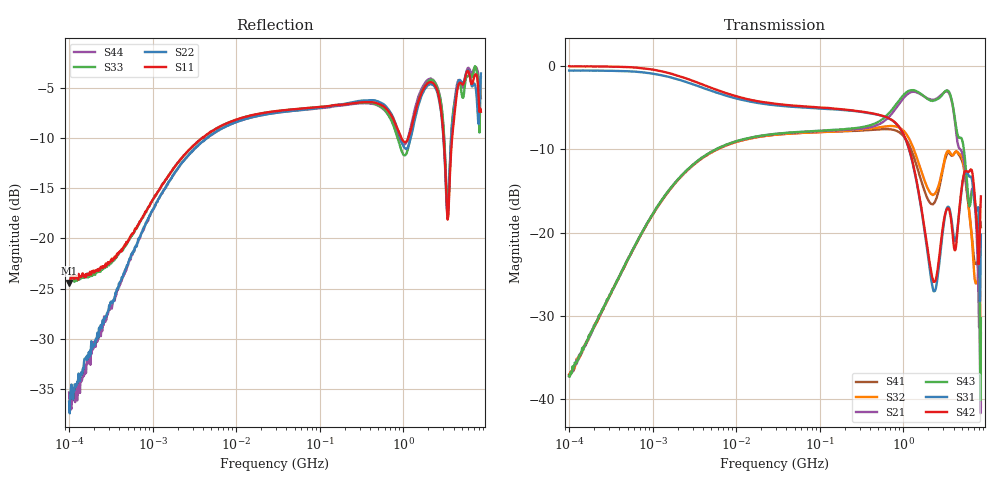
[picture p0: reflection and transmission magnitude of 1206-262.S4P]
!Agilent Technologies,E5071C,MY46110495,A.10.06
!Date: Tue Jun 06 11:35:06 2017
!Data & Calibration Information:
!Freq	S11:SOLT4(ON)	S12:SOLT4(ON)	S13:SOLT4(ON)	S14:SOLT4(ON)
!	S21:SOLT4(ON)	S22:SOLT4(ON)	S23:SOLT4(ON)	S24:SOLT4(ON)
!	S31:SOLT4(ON)	S32:SOLT4(ON)	S33:SOLT4(ON)	S34:SOLT4(ON)
!	S41:SOLT4(ON)	S42:SOLT4(ON)	S43:SOLT4(ON)	S44:SOLT4(ON)
!PortZ  Port1:50+j0  Port2:50+j0  Port3:50+j0  Port4:50+j0
!Above PortZ is port z conversion or system Z0 setting when saving the data.
!When reading, reference impedance value at option line is always used.
# Hz S dB R 50
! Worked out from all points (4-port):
!   801 points, 100 kHz to 8.5 GHz, reference 50 ohm
!   strongest paths, dB at 100 kHz, 1.721 MHz, 29.51 MHz, 502.3 MHz, 8.5 GHz:
!     S42: -0.1, -1.0, -4.6, -5.9, -15.7
!     S31: -0.6, -1.5, -4.8, -5.9, -20.2
!     S43: -37.2, -14.4, -8.2, -6.7, -30.3
!     S21: -37.2, -14.4, -8.2, -7.1, -32.0
!     S32: -37.2, -14.5, -8.3, -7.4, -40.8
!     S41: -37.0, -14.5, -8.3, -7.7, -19.4
!   lowest |S11| = -24.4 dB at 100 kHz (marker M1), VSWR 1.13, Z = 56.2 + j1.36 ohm
!   |S11| at or under -10 dB: start of sweep to 3.936 MHz; 947.3 MHz to 1.151 GHz (203.9 MHz wide, 19.4 % of centre); 3.04 GHz to 3.848 GHz (808.2 MHz wide, 23.5 % of centre)
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100000  -24.43 11.5  -36.92 87.1  -0.57 -0.6  -37.26 -91.7
        -37.24 88.5  -36.26 63.8  -37.54 -93.0  -0.09 -0.7
        -0.59 -0.7  -37.21 -93.0  -24.49 15.9  -37.09 88.0
        -37.01 -92.0  -0.06 -0.7  -37.17 87.9  -35.34 74.8
4284339  -9.78 28.5  -10.77 33.9  -2.76 -12.3  -10.83 -146.9
         -10.77 33.9  -10.16 33.5  -10.84 -146.8  -2.41 -13.2
         -2.77 -12.4  -10.84 -146.7  -9.79 28.5  -10.76 33.8
         -10.82 -146.6  -2.39 -13.3  -10.75 33.8  -10.12 33.8
1.316504e9  -8.22 68.2  -3.13 2.0  -11.98 -111.2  -10.73 61.7
            -3.13 2.1  -8.91 69.4  -9.84 59.0  -11.87 -111.8
            -11.98 -111.1  -9.84 59.0  -8.51 72.2  -2.94 0.1
            -10.73 61.8  -11.86 -111.8  -2.93 0.1  -7.83 71.2
2.609641e9  -5.56 82.7  -3.82 -14.4  -24.93 104.7  -15.23 59.2
            -3.82 -14.4  -5.77 83.9  -14.57 47.8  -24.08 108.9
            -24.95 105.0  -14.57 47.8  -5.21 83.4  -3.97 -14.1
            -15.24 59.2  -24.04 109.2  -3.97 -14.1  -5.14 83.0
4.787885e9  -4.49 -99.0  -10.00 -55.4  -16.55 116.4  -10.91 -40.8
            -10.01 -55.3  -4.24 -101.1  -10.65 -44.2  -16.39 114.7
            -16.55 116.5  -10.65 -44.1  -4.57 -105.6  -8.67 -53.2
            -10.89 -40.6  -16.36 114.8  -8.67 -53.2  -4.40 -99.0
6.738951e9  -4.56 10.3  -14.77 -49.5  -14.04 3.3  -21.19 -175.5
            -14.73 -49.4  -4.87 4.4  -21.66 -171.0  -12.93 4.7
            -14.04 3.6  -21.70 -170.8  -3.94 11.4  -15.02 -46.9
            -21.13 -175.2  -12.93 5.0  -14.98 -46.7  -3.60 10.5
8.5e9  -7.40 112.9  -31.82 55.8  -20.24 40.1  -19.37 35.6
       -32.05 57.1  -3.59 128.0  -40.86 95.2  -15.68 24.3
       -20.24 40.1  -40.84 95.6  -3.97 130.0  -30.24 26.2
       -19.35 35.9  -15.66 24.6  -30.26 25.3  -6.05 100.4
